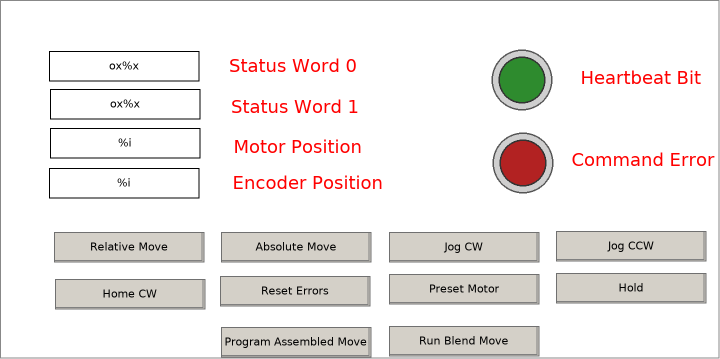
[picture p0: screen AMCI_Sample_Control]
VISUALIZATION AMCI_Sample_Control  // 720x359
    Rectangle (49,51 150x30), "ox%x", text variable: SMD23K_data.iStatus0
    Rectangle (50,89 150x30), "ox%x", text variable: SMD23K_data.iStatus1
    Rectangle (50,128 150x30), "%i", text variable: SMD23K_data.iMotorPos
    Rectangle (49,168 150x30), "%i", text variable: SMD23K_data.iEncPos
    Label (218,51 150x30), "Status Word 0"
    Label (220,92 150x30), "Status Word 1"
    Label (223,132 150x30), "Motor Position"
    Label (233,168 150x30), "Encoder Position"
    Lamp1 (487,45 70x70), variable: SMD23K_data.iStatus1.11, style: Lamp-Lamp1-Green
    Label (566,63 150x30), "Heartbeat Bit"
    Lamp1 (488,128 70x70), variable: SMD23K_data.iStatus0.12, style: Lamp-Lamp1-Red
    Label (568,145 150x30), "Command Error"
    Button (54,232 150x30), "Relative Move", colour toggle: b_relative_move_1_button
        OnMouseClick: toggle b_relative_move_1_button
    Button (221,232 150x30), "Absolute Move", colour toggle: b_absolute_move_1_button
        OnMouseClick: toggle b_absolute_move_1_button
    Button (389,232 150x30), "Jog CW", colour toggle: b_jog_cw_1_button
        OnMouseClick: toggle b_jog_cw_1_button
    Button (556,231 150x30), "Jog CCW", colour toggle: b_jog_ccw_1_button
        OnMouseClick: toggle b_jog_ccw_1_button
    Button (55,279 150x30), "Home CW", colour toggle: b_home_CW_button
        OnMouseClick: toggle b_home_CW_button
    Button (220,276 150x30), "Reset Errors", colour toggle: b_reset_errors_button
        OnMouseClick: toggle b_reset_errors_button
    Button (389,274 150x30), "Preset Motor", colour toggle: b_preset_button
        OnMouseClick: toggle b_preset_button
    Button (556,273 150x30), "Hold", colour toggle: b_hold_button
        OnMouseClick: toggle b_hold_button
    Button (221,327 150x30), "Program Assembled Move", colour toggle: b_program_assembled_move
        OnMouseClick: toggle b_program_assembled_move
    Button (389,326 150x30), "Run Blend Move", colour toggle: b_run_blend_move
        OnMouseClick: toggle b_run_blend_move
END_VISUALIZATION
